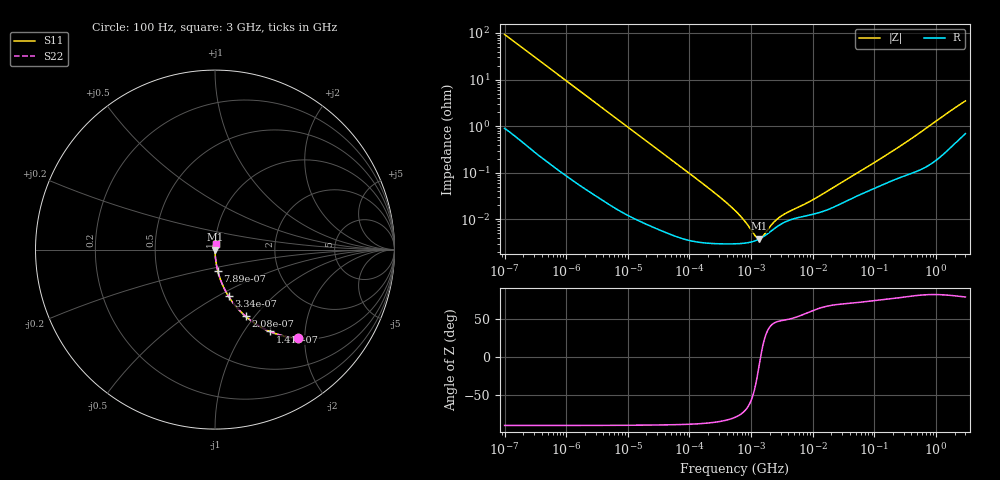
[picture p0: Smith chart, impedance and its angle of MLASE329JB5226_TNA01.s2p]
! MLASE329JB5226_TNA01  S-PARAMETER MODEL  ( Standard Model )
! Model Generated by TAIYO YUDEN Corporation (http://www.ty-top.com)
! Version 1.0
! TAIYO YUDEN Control No. 220601
! Copyright(c) 2008 TAIYO YUDEN CO.,LTD. All Rights Reserved.
! Product Description (link to TY-COMPAS)
! https://ds.yuden.co.jp/TYCOMPAS/or/detail?pn=MLASE329JB5226MTNA01&u=M
! Products Name : Multilayer Ceramic Capacitors
! Characteristics :
!  Capacitance : 22 [uF] , Rated Voltage : 16 [V] , TCC : X5R
!  Case Size : 3.2 x 2.5 / 0.126 x 0.098 [mm/inch] , Thickness : 0.85 / 0.033 [mm/inch]
!  (Conditions: Temperature = 25 [degC] , DC Bias Voltage = 0 [V])
! External Node Assignments :
!  1  o---| |---o  2
! GND o---------o GND
! Frequency Range : 100Hz  -  3GHz  [ 401 STEP ]
# MHZ S RI R 50
! Freq[MHz].  S11 Real  S11 Imag  S21 Real  S21 Imag  S12 Real  S12 Imag  S22 Real  S22 Imag
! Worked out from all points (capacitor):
!   401 points, 100 Hz to 3 GHz, reference 50 ohm
!   read as one part in series: C = 17.1 uF near 109 Hz
!   lowest |Z| = 3.84 mohm at 1.352 MHz (marker M1)
!   series resonance near 1.426 MHz, so ESL is about 730 pH
!   S11 on the Smith chart (normalised r, x): 100 Hz: 1.02, -1.86; 141 Hz: 1.01, -1.32; 208 Hz: 1.01, -0.90; 334 Hz: 1.01, -0.56; 789 Hz: 1.00, -0.24; 3 GHz: 1.01, +0.07
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0.0001  0.4647 -0.494  0.5353 0.494  0.5353 0.494  0.4647 -0.494
0.000141  0.3061 -0.4561  0.6939 0.4561  0.6939 0.4561  0.3061 -0.4561
0.000208  0.1709 -0.3717  0.8291 0.3717  0.8291 0.3717  0.1709 -0.3717
0.000334  0.0753 -0.2594  0.9247 0.2594  0.9247 0.2594  0.0753 -0.2594
0.000513  0.034 -0.1767  0.966 0.1767  0.966 0.1767  0.034 -0.1767
0.000789  0.0151 -0.1175  0.9849 0.1175  0.9849 0.1175  0.0151 -0.1175
0.001788  0.00329 -0.0527  0.9967 0.0527  0.9967 0.0527  0.00329 -0.0527
0.005476  0.000494 -0.0174  0.9995 0.0174  0.9995 0.0174  0.000494 -0.0174
0.031977  6.9e-05 -0.00301  0.9999 0.00301  0.9999 0.00301  6.9e-05 -0.00301
0.231582  3.05e-05 -0.00041  1 0.00041  1 0.00041  3.05e-05 -0.00041
0.388167  2.98e-05 -0.000233  1 0.000233  1 0.000233  2.98e-05 -0.000233
0.547723  2.99e-05 -0.000152  1 0.000152  1 0.000152  2.99e-05 -0.000152
0.709116  3.04e-05 -0.000104  1 0.000104  1 0.000104  3.04e-05 -0.000104
0.772864  3.07e-05 -8.97e-05  1 8.97e-05  1 8.97e-05  3.07e-05 -8.97e-05
1.352413  3.77e-05 -7.11e-06  1 7.11e-06  1 7.11e-06  3.77e-05 -7.11e-06
2.579298  6.83e-05 7.06e-05  0.9999 -7.06e-05  0.9999 -7.06e-05  6.83e-05 7.06e-05
3.79959  9.14e-05 0.000105  0.9999 -0.000105  0.9999 -0.000105  9.14e-05 0.000105
9.794414  0.000127 0.000225  0.9999 -0.000225  0.9999 -0.000225  0.000127 0.000225
175.1444  0.000646 0.00256  0.9994 -0.00256  0.9994 -0.00256  0.000646 0.00256
414.2403  0.00101 0.0055  0.999 -0.0055  0.999 -0.0055  0.00101 0.0055
1950.712  0.0046 0.0234  0.9954 -0.0234  0.9954 -0.0234  0.0046 0.0234
3000  0.008 0.0336  0.992 -0.0336  0.992 -0.0336  0.008 0.0336
